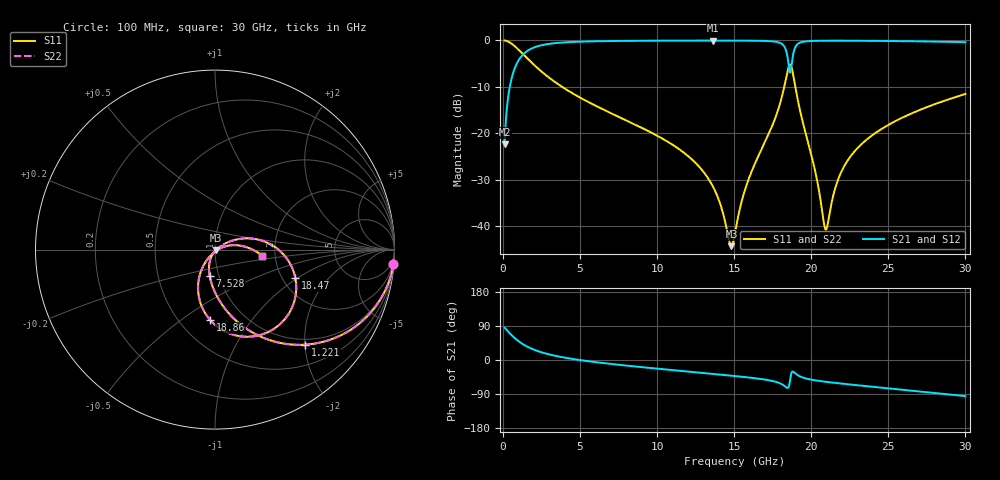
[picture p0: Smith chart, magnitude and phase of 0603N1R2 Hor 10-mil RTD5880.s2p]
# GHz S MA R 50
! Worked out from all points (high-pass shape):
!   3201 points, 100 MHz to 30 GHz, reference 50 ohm
!   highest |S21| = -0.05 dB at 13.62 GHz (marker M1); lowest = -22.4 dB at 100 MHz (marker M2)
!   |S21| within 3 dB of the highest: 1.299 GHz to 18.43 GHz (17.13 GHz wide, 174 % of centre); 18.82 GHz to end of sweep
!   lowest |S11| = -44.3 dB at 14.82 GHz (marker M3), VSWR 1.01, Z = 50.4 - j0.415 ohm
!   |S11| at or under -10 dB: 3.82 GHz to 18.25 GHz (14.43 GHz wide, 131 % of centre); 18.96 GHz to end of sweep
!   |S22| runs from -44.3 to 0.0 dB; largest |S21 - S12| = 0
!   S11 on the Smith chart (normalised r, x): 100 MHz: 1, -25; 1.221 GHz: 0.88, -2.01; 7.528 GHz: 0.90, -0.27; 18.47 GHz: 2.35, -0.96; 18.86 GHz: 0.70, -0.65; 30 GHz: 1.71, -0.12
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0.1  0.997 -4.6  0.07604 85.3  0.07604 85.3  0.997 -4.6
0.5204688  0.9293 -23.1  0.3687 66.8  0.3687 66.8  0.9293 -23.1
1.22125  0.7307 -46.5  0.6817 43.5  0.6817 43.5  0.7307 -46.5
2.632156  0.4411 -71.1  0.8957 18.7  0.8957 18.7  0.4411 -71.1
5.089563  0.2369 -90.1  0.9688 -0.8  0.9688 -0.8  0.2369 -90.1
7.528281  0.1493 -101.5  0.9854 -12.7  0.9854 -12.7  0.1493 -101.5
10.06978  0.09251 -110.6  0.9916 -23.1  0.9916 -23.1  0.09251 -110.6
13.62041  0.02654 -115.1  0.9942 -36.6  0.9942 -36.6  0.02654 -115.1
14.81641  0.006064 -42.7  0.9937 -41.4  0.9937 -41.4  0.006064 -42.7
15.05  0.008404 -0.6  0.9935 -42.3  0.9935 -42.3  0.008404 -0.6
15.84422  0.02904 29.7  0.9921 -45.7  0.9921 -45.7  0.02904 29.7
18.00262  0.217 16.4  0.9336 -62.1  0.9336 -62.1  0.217 16.4
18.46981  0.475 -19.5  0.645 -73.8  0.645 -73.8  0.475 -19.5
18.67537  0.5393 -61.7  0.4783 -40.2  0.4783 -40.2  0.5393 -61.7
18.86225  0.3919 -94.1  0.7557 -31.8  0.7557 -31.8  0.3919 -94.1
19.30141  0.1663 -120.8  0.9489 -43.9  0.9489 -43.9  0.1663 -120.8
20.03956  0.05507 -127.8  0.9847 -52.1  0.9847 -52.1  0.05507 -127.8
20.96459  0.009152 -49.3  0.9907 -57.6  0.9907 -57.6  0.009152 -49.3
21.60931  0.02744 12.0  0.9912 -60.7  0.9912 -60.7  0.02744 12.0
22.27272  0.0482 17.1  0.9908 -63.6  0.9908 -63.6  0.0482 17.1
25.01978  0.1232 11.4  0.9842 -74.9  0.9842 -74.9  0.1232 11.4
30  0.2645 -7.3  0.9548 -95.3  0.9548 -95.3  0.2645 -7.3
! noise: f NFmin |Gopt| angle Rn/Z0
0.1  0.002092  0.9883  0.3377  0.0408
3.417  0.004065  0.8114  10.2  0.004461
6.743  0.006809  0.7823  19.43  0.006239
10.06  0.009387  0.7681  28.56  0.007747
13.39  0.01222  0.7657  37.56  0.009521
16.7  0.01867  0.8066  46.32  0.01701
20.03  0.02402  0.8208  55.2  0.02213
23.35  0.01933  0.7535  63.44  0.01154
26.67  0.02145  0.7503  71.51  0.01152
30  0.02417  0.7539  79.35  0.01191
